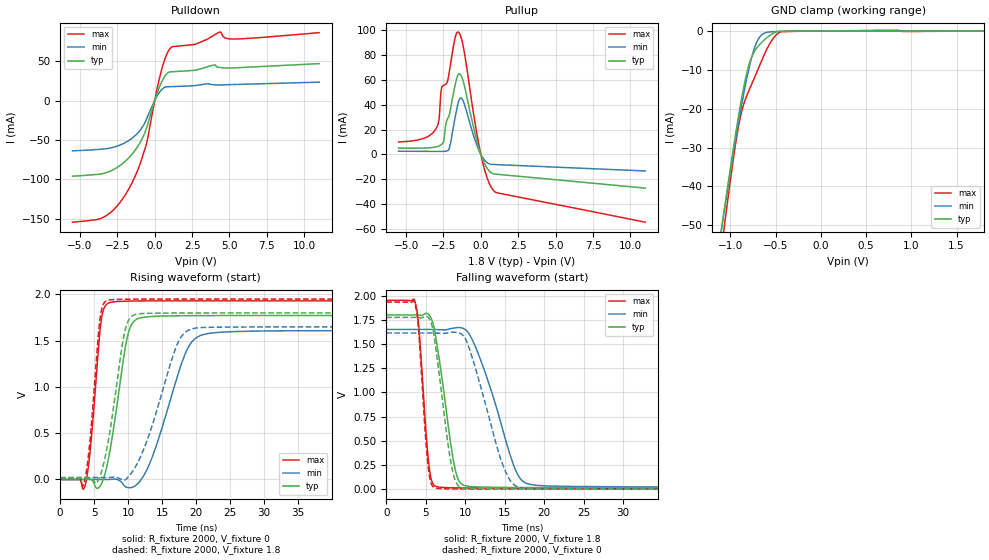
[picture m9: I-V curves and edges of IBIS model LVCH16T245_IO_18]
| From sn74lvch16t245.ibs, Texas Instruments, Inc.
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[Model]   LVCH16T245_IO_18
Model_type  I/O
Vinl=0.5775
Vinh=1.2675
Enable   Active-Low
Vref =   0
Rref =   2000
Cref =   15p
Vmeas =   0.9
| variable   typ   min   max
C_comp   6.46pF   5.54pF   7.47pF
| C_pullup   10.93pF   6.91pF   16.41pF
| C_pulldown   10.27pF   6.93pF   16.47pF
| C_tri-state   6.46pF   5.54pF   7.47pF
[Temperature Range]   40   100   -40
| Ambient temperature   25   85   -40
[Voltage range]   1.8   1.65   1.95
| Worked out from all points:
|   slope of the pulldown table from 0 to 0.27 V, typ, clamps not added: 18.2 ohm
|   slope of the pullup table from 0 to 0.27 V, typ, clamps not added: 34.2 ohm
|   GND clamp passes 1 mA (typ) near -0.56 V on its own axis
|   rising waveform, R_fixture 2000, V_fixture 0: 20-80 % time 2.14ns typ, 4.1ns min, 1.27ns max; typ from 0 V to 1.77 V
|   falling waveform, R_fixture 2000, V_fixture 1.8: 20-80 % time 1.83ns typ, 3.71ns min, 994ps max; typ from 1.8 V to 0.015 V
|   rising waveform, R_fixture 2000, V_fixture 1.8: 20-80 % time 2.14ns typ, 4.14ns min, 1.26ns max; typ from 0.015 V to 1.8 V
|   falling waveform, R_fixture 2000, V_fixture 0: 20-80 % time 1.69ns typ, 3.31ns min, 941ps max; typ from 1.77 V to 0 V
[GND Clamp]
| LVCH16T245_IO_18
|   Voltage   I(typ)   I(min)   I(max)
-5.5V     -898.4mA   -832.7mA   -1.017A
-1.11V    -52.9mA    -52.49mA   -58.08mA
-1.08V    -47.95mA   -47.91mA   -52.49mA
-1.05V    -43.06mA   -43.39mA   -47.01mA
-910mV    -21.73mA   -23.39mA   -24.4mA
-835mV    -12.36mA   -13.93mA   -17.58mA
-785mV    -7.908mA   -8.545mA   -14.71mA
-735mV    -5.261mA   -4.378mA   -12.02mA
-645mV    -2.699mA   -814.8uA   -7.048mA
-520mV    -490.8uA   -164.8uA   -1.664mA
-430mV    -95.06uA   -91.61uA   -151.8uA
1.8V      25.08pA    236.4nA    -4.713nA
[Pulldown]
| LVCH16T245_IO_18
|   Voltage   I(typ)   I(min)   I(max)
-5.5V     -95.82mA   -63.67mA   -154.2mA
-3.315V   -91.75mA   -61.14mA   -146.8mA
-1.75V    -72.89mA   -50.79mA   -112.6mA
-1.13V    -58mA      -41.04mA   -87.84mA
-600mV    -37.68mA   -25.69mA   -57.96mA
405mV     21.1mA     12.54mA    35.05mA
770mV     33.15mA    17.47mA    57.09mA
1.105V    36.55mA    17.72mA    67.48mA
2.715V    38.65mA    19.07mA    71.4mA
4.38V     42.01mA    19.88mA    86.86mA
5.235V    41.5mA     20.34mA    78.05mA
11V       46.88mA    23.37mA    86.19mA
[Pullup]
| LVCH16T245_IO_18
|   Voltage   I(typ)   I(min)   I(max)
-5.5V     5.088mA    2.627mA    10.09mA
-3.805V   5.165mA    2.515mA    13.04mA
-2.98V    6.16mA     2.455mA    21.15mA
-2.8V     6.846mA    2.441mA    28.18mA
-2.625V   8.108mA    2.443mA    53.57mA
-2.135V   31.01mA    4.02mA     64.57mA
-1.74V    54.87mA    28.55mA    92.96mA
-1.515V   64.43mA    41.57mA    98.64mA
-1.185V   59.29mA    43.25mA    87.57mA
35mV      -1.184mA   -766.3uA   -1.908mA
875mV     -15.72mA   -8.085mA   -29.46mA
11V       -27.14mA   -13.3mA    -54.59mA
[Ramp]
| LVCH16T245_IO_18
| variable   typ   min   max
dV/dt_r   1.12/2.28E-09   1.02/4.35E-09   1.22/1.35E-09
dV/dt_f   1.08/1.85E-09   0.99/3.76E-09   1.17/1.00E-09
R_load = 2000
[Rising Waveform]
| LVCH16T245_IO_18
R_fixture =   2000
C_fixture =   0
L_fixture =   0
V_fixture =   0
V_fixture_min = 0
V_fixture_max = 0
|   Time   V(typ)   V(min)   V(max)
0s        294.6pV    9.345nV    2.358nV
3.7ns     -78.01uV   -62.25nV   -57.67mV
4.48ns    4.278mV    335.2nV    355.3mV
5.975ns   -61.58mV   -29.48uV   1.679V
7.025ns   192.7mV    -193.7uV   1.903V
9.79ns    1.505V     -84.7mV    1.927V
11.32ns   1.734V     -52.89mV   1.929V
18.43ns   1.77V      1.362V     1.931V
20.25ns   1.771V     1.541V     1.931V
50ns      1.772V     1.61V      1.931V
[Falling Waveform]
| LVCH16T245_IO_18
R_fixture =   2000
C_fixture =   0
L_fixture =   0
V_fixture =   1.8
V_fixture_min = 1.65
V_fixture_max = 1.95
|   Time   V(typ)   V(min)   V(max)
0s        1.8V       1.65V      1.95V
3.685ns   1.8V       1.65V      1.922V
4.125ns   1.797V     1.65V      1.669V
5.37ns    1.805V     1.65V      272.5mV
6.225ns   1.588V     1.649V     31.32mV
8.56ns    270.5mV    1.664V     14.05mV
9.785ns   41.44mV    1.659V     12.63mV
11.54ns   23.28mV    1.421V     11.61mV
17.61ns   16.76mV    65.62mV    10.39mV
50ns      14.81mV    21.77mV    9.836mV
[Rising Waveform]
| LVCH16T245_IO_18
R_fixture =   2000
C_fixture =   0
L_fixture =   0
V_fixture =   1.8
V_fixture_min = 1.65
V_fixture_max = 1.95
|   Time   V(typ)   V(min)   V(max)
0s        14.75mV    21.42mV    9.831mV
3.53ns    14.69mV    21.42mV    -38.62mV
4.355ns   18.59mV    21.42mV    395.9mV
5.825ns   26.99mV    21.4mV     1.712V
6.8ns     301.3mV    21.34mV    1.931V
9.395ns   1.557V     -9.303mV   1.948V
10.81ns   1.777V     104mV      1.949V
17.07ns   1.799V     1.431V     1.95V
18.85ns   1.8V       1.612V     1.95V
50ns      1.8V       1.65V      1.95V
[Falling Waveform]
| LVCH16T245_IO_18
R_fixture =   2000
C_fixture =   0
L_fixture =   0
V_fixture =   0
V_fixture_min = 0
V_fixture_max = 0
|   Time   V(typ)   V(min)   V(max)
0s        1.774V     1.613V     1.932V
3.645ns   1.774V     1.613V     1.911V
4.085ns   1.772V     1.613V     1.653V
5.26ns    1.78V      1.613V     265.6mV
6.1ns     1.554V     1.612V     15.48mV
8.17ns    282.7mV    1.62V      2.587mV
9.44ns    17.88mV    1.605V     1.756mV
14.68ns   1.562mV    269.7mV    708.3uV
16.49ns   1.169mV    29.26mV    545.7uV
50ns      53.37uV    210uV      5.562uV
